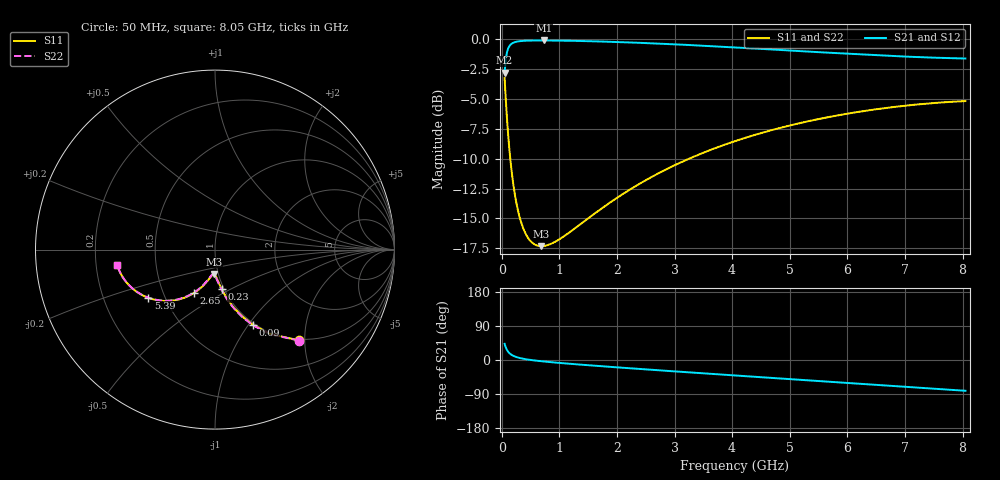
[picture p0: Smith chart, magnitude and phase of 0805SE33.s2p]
! AVX Thin Film Operation		Date: August 2001
! Description: Accu-P® Series, Thin Film, SMD, RF Capacitor
! Part Number: 08053J330FBT
! 50 MHz  -  8.05 GHz
! Serial Measurements
# mhz S db R 50
!	S11		S21		S12		S22
!	dB	Phase	dB	Phase	dB	Phase	dB	Phase
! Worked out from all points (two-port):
!   401 points, 50 MHz to 8.05 GHz, reference 50 ohm
!   highest |S21| = -0.08 dB at 730 MHz (marker M1); lowest = -2.8 dB at 50 MHz (marker M2)
!   |S21| within 3 dB of the highest: start of sweep to end of sweep
!   lowest |S11| = -17.3 dB at 690 MHz (marker M3), VSWR 1.32, Z = 47.6 - j13.2 ohm
!   |S11| at or under -10 dB: 148.6 MHz to 3.249 GHz (3.101 GHz wide, 183 % of centre)
!   |S22| runs from -17.3 to -3.2 dB; largest |S21 - S12| = 0
!   S11 on the Smith chart (normalised r, x): 50 MHz: 0.98, -1.88; 90 MHz: 0.98, -1.06; 230 MHz: 0.97, -0.45; 2.65 GHz: 0.71, -0.37; 5.39 GHz: 0.40, -0.28; 8.05 GHz: 0.29, -0.07
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50  -3.24 -47.2  -2.79 42.7  -2.79 42.7  -3.24 -47.3
90  -6.53 -63.1  -1.10 26.7  -1.10 26.7  -6.53 -63.4
110  -7.89 -67.8  -0.77 22.0  -0.77 22.0  -7.89 -68.1
130  -9.06 -71.2  -0.58 18.5  -0.58 18.5  -9.06 -71.6
150  -10.07 -73.9  -0.45 15.9  -0.45 15.9  -10.07 -74.3
190  -11.75 -77.7  -0.30 11.9  -0.30 11.9  -11.75 -78.3
230  -13.04 -80.4  -0.22 9.2  -0.22 9.2  -13.04 -81.1
310  -14.88 -84.1  -0.15 5.4  -0.15 5.4  -14.88 -84.9
410  -16.23 -87.1  -0.11 2.3  -0.11 2.3  -16.23 -88.1
530  -17.04 -89.8  -0.09 -0.4  -0.09 -0.4  -17.04 -90.8
690  -17.32 -92.6  -0.08 -3.3  -0.08 -3.3  -17.32 -93.7
730  -17.31 -93.2  -0.08 -3.9  -0.08 -3.9  -17.31 -94.3
970  -16.84 -96.7  -0.09 -7.3  -0.09 -7.3  -16.84 -97.7
1390  -15.40 -101.9  -0.13 -12.5  -0.13 -12.5  -15.40 -102.8
2030  -13.18 -109.3  -0.22 -19.7  -0.22 -19.7  -13.18 -109.9
2650  -11.40 -116.0  -0.33 -26.4  -0.33 -26.4  -11.40 -116.5
2730  -11.20 -116.8  -0.35 -27.2  -0.35 -27.2  -11.20 -117.3
3350  -9.79 -123.3  -0.49 -33.7  -0.49 -33.7  -9.79 -123.7
4050  -8.52 -130.5  -0.67 -40.8  -0.67 -40.8  -8.52 -130.9
5390  -6.78 -144.0  -1.03 -54.3  -1.03 -54.3  -6.78 -144.3
6730  -5.70 -157.5  -1.38 -67.7  -1.38 -67.7  -5.70 -157.6
8050  -5.16 -171.0  -1.60 -81.2  -1.60 -81.2  -5.16 -171.1
